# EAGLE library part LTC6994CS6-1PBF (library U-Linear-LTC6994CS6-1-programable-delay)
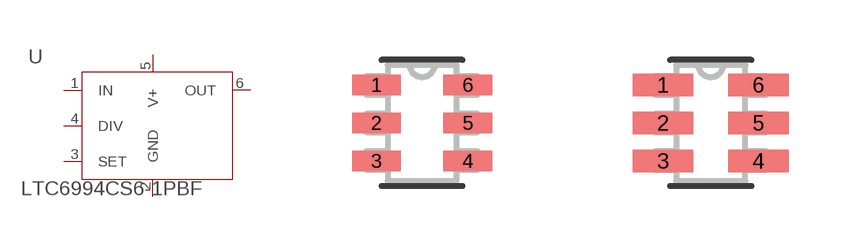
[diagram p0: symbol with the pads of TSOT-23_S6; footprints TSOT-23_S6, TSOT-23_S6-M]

Designator prefix U

## LTC6994CS6-1PBF (MFR: Linear Technology; MPN: LTC6994-1; VALUE: LTC6994-1)  [TSOT-23_S6]
1  IN  in
2  GND  pwr
3  SET  in
4  DIV  in
5  V+  pwr
6  OUT  out

## LTC6994CS6-1PBFTSOT-23_S6-M (MANUFACTURER_PART_NUMBER: LTC6994CS61#PBF; VENDOR: Linear Technology)  [TSOT-23_S6-M]
Pads as for TSOT-23_S6

## LTC6994CS6-1PBFTSOT-23_S6-L (MANUFACTURER_PART_NUMBER: LTC6994CS61#PBF; VENDOR: Linear Technology)  [TSOT-23_S6-L]
Pads as for TSOT-23_S6

## Footprint TSOT-23_S6 (pad centres in mm)
smd 1.219 x 0.508: 1 -1.143,0.95; 2 -1.143,0; 3 -1.143,-0.95; 4 1.143,-0.95; 5 1.143,0; 6 1.143,0.95

## Footprint TSOT-23_S6-M (pad centres in mm)
smd 1.524 x 0.559: 1 -1.194,0.95; 2 -1.194,0; 3 -1.194,-0.95; 4 1.194,-0.95; 5 1.194,0; 6 1.194,0.95

## Footprint TSOT-23_S6-L (pad centres in mm)
smd 0.914 x 0.457: 1 -1.092,0.95; 2 -1.092,0; 3 -1.092,-0.95; 4 1.092,-0.95; 5 1.092,0; 6 1.092,0.95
